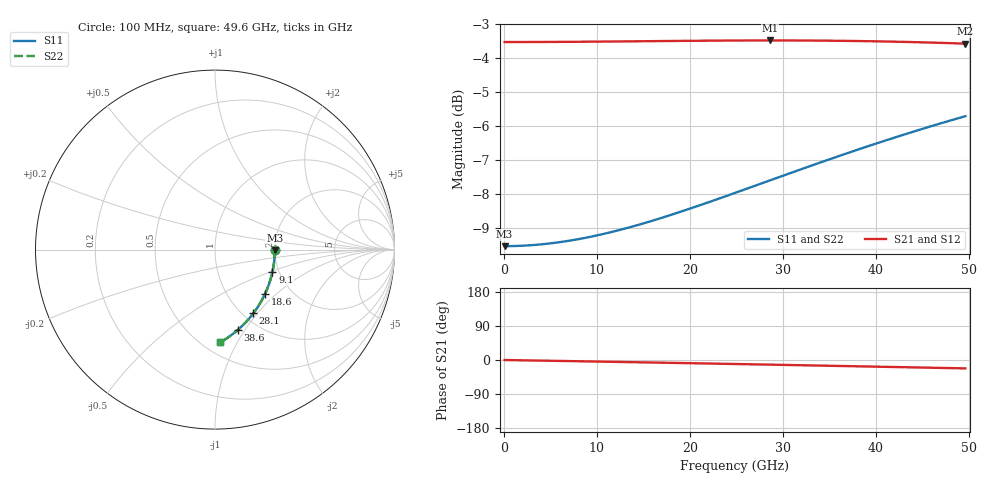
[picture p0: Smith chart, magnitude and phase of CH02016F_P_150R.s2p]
# GHz S RI R 150
! S-Parameters data
! Freq  reS11  imS11  reS21  imS21  reS12  imS12  reS22  imS22
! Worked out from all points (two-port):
!   100 points, 100 MHz to 49.6 GHz, reference 150 ohm
!   highest |S21| = -3.48 dB at 28.6 GHz (marker M1); lowest = -3.6 dB at 49.6 GHz (marker M2)
!   |S21| within 3 dB of the highest: start of sweep to end of sweep
!   lowest |S11| = -9.5 dB at 100 MHz (marker M3), VSWR 2.00, Z = 300 - j0.952 ohm
!   |S11| at or under -10 dB: nowhere
!   |S22| runs from -9.5 to -5.7 dB; largest |S21 - S12| = 0
!   S11 on the Smith chart (normalised r, x): 100 MHz: 2.00, -0.01; 9.1 GHz: 1.84, -0.53; 18.6 GHz: 1.47, -0.85; 28.1 GHz: 1.11, -0.95; 38.6 GHz: 0.81, -0.93; 49.6 GHz: 0.60, -0.85
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0.1  0.3333 -0.00141  0.6667 -0.000475  0.6667 -0.000475  0.3333 -0.00141
2.1  0.3326 -0.0296  0.6666 -0.00997  0.6666 -0.00997  0.3326 -0.0296
4.1  0.3305 -0.0577  0.6665 -0.0195  0.6665 -0.0195  0.3305 -0.0577
6.1  0.327 -0.0855  0.6664 -0.0291  0.6664 -0.0291  0.327 -0.0855
8.6  0.3209 -0.12  0.6661 -0.0411  0.6661 -0.0411  0.3209 -0.12
9.1  0.3194 -0.1268  0.666 -0.0435  0.666 -0.0435  0.3194 -0.1268
10.6  0.3145 -0.147  0.6657 -0.0508  0.6657 -0.0508  0.3145 -0.147
12.6  0.3069 -0.1736  0.6653 -0.0606  0.6653 -0.0606  0.3069 -0.1736
14.6  0.2982 -0.1996  0.6647 -0.0705  0.6647 -0.0705  0.2982 -0.1996
16.6  0.2883 -0.2249  0.6639 -0.0805  0.6639 -0.0805  0.2883 -0.2249
18.6  0.2774 -0.2495  0.663 -0.0906  0.663 -0.0906  0.2774 -0.2495
21.6  0.2592 -0.285  0.6612 -0.106  0.6612 -0.106  0.2592 -0.285
25.1  0.2355 -0.324  0.6585 -0.1241  0.6585 -0.1241  0.2355 -0.324
28.1  0.2134 -0.3552  0.6555 -0.1398  0.6555 -0.1398  0.2134 -0.3552
28.6  0.2096 -0.3602  0.6549 -0.1424  0.6549 -0.1424  0.2096 -0.3602
31.1  0.1899 -0.3843  0.6519 -0.1555  0.6519 -0.1555  0.1899 -0.3843
33.1  0.1736 -0.4026  0.6491 -0.166  0.6491 -0.166  0.1736 -0.4026
35.6  0.1525 -0.424  0.6451 -0.1791  0.6451 -0.1791  0.1525 -0.424
38.6  0.1265 -0.4478  0.6398 -0.1947  0.6398 -0.1947  0.1265 -0.4478
41.6  0.0998 -0.4695  0.6337 -0.2101  0.6337 -0.2101  0.0998 -0.4695
45.6  0.0637 -0.4953  0.6245 -0.2302  0.6245 -0.2302  0.0637 -0.4953
49.6  0.0271 -0.5176  0.6142 -0.2497  0.6142 -0.2497  0.0271 -0.5176
